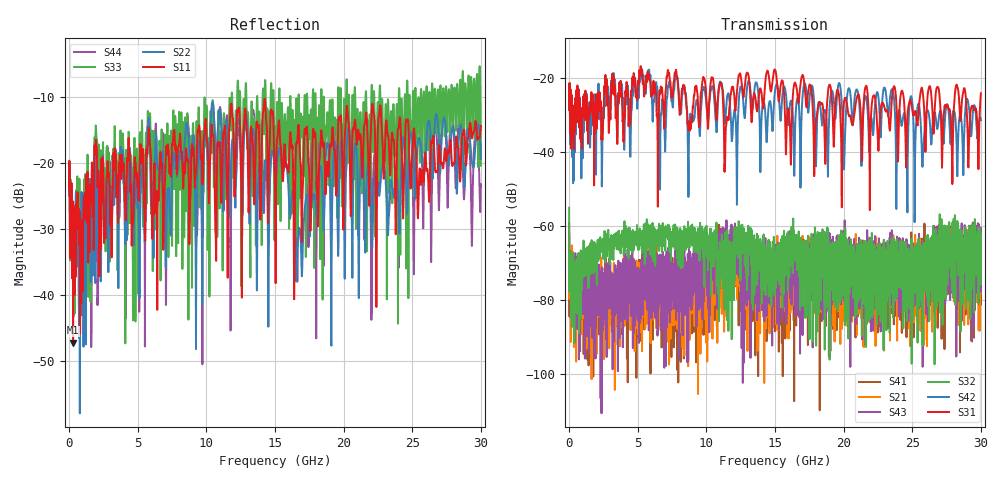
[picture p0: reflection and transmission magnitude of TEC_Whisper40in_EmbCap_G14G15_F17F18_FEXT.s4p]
! Tyco Electronics
! F17F18-G14G15_FEXT
!! PART DESCRIPTION: Whisper 40in Megtron 6 VLP-HVLP-VLP Channel, Embedded Capactior Connecter at one end, bulkhead 2.4mm test pts
!! MODEL DESCRIPTION: System 4-port S-parameter
!! MODEL STATUS: Measured
!! MODEL GEOMETRY: Channel Model
!! MODEL FREQUENCY RANGE: DC to 30.000 GHz in 10.000 MHz frequency steps
!! MODEL EDGE RATE LIMITATION: 12.500 ps (Using conservative 0.5/Fmax rule of thumb)
!! TIME-DOMAIN TRANSFORM CAUTIONS:
!! 1.) Do not simulate transient edge rates faster than the number listed above.  Edge rates faster than this number
!!  contain significant spectral content at frequencies above the model's highest frequency.
!! 2.) Even when simulating edge rates that are slower than the number listed above, be aware that the best time
!!  resolution possible with a direct iFFT is (1 / 2Fmax).  As a result, time resolution is typically not adequate
!!  for most time-domain simulations unless tricks such as windowing are used to minimize leakage and aliasing.
!! 3.) Because the model has a uniform frequency step, a direct iFFT will result in an impulse that that has a time
!!  length given by either (1 / Fstep) or (1 / 2Fstep), depending on the transform being used.  Care has been taken
!!  in selecting the frequency step to ensure a settled impulse response for the model.  Therefore, convolution with
!!  the model's impulse response should present no issues.  However, if directly concatenating s-parameter models
!!  in the frequency domain a user must either interpolate necessary interim frequencies or complete impulse response
!!  zero-padding.  Impulse response zero-padding is more difficult, but more accurate.
!! PORT DEFINITIONS:
!! Port  1  ----->  Side A  F17  G14  Side B  <-----  Port  2
!! Port  3  ----->  Side A  F18  G15  Side B  <-----  Port  4
! Point-to-Point link (differential)  !
! Connectors:  !
!  1: STRADA Whisper  !
! Materials:  !
!  Backplane: Megtron-6 HVLP  !
!  Daughtercard: Megtron-6 VLP  !
! Stack-up:  !
!  Backplane: 20 layers, 200mil thick  !
!  Daughtercard: 14 layers, 110mil thick  !
! Trace Length:  !
!  Backplane: 30in  !
!  Daightercards: 5in  !
! Trace Width:  !
!  Backplane: 7-9-7 mils  !
!  Daughtercards: 6-9-6 mils  !
! Geometry:  !
!  Backplane: Stripline  !
!  Daughtercards: Stripline  !
! Freq. Range: 0 GHz - 30 GHz  !
! Note1: non-mixed-mode s-parameters  !
! Note2: channel includes 2.4mm test points  !
! Touchstone data
! Created: 02-Jul-2013 by IdEM R2011 (7.0.3)
# Hz S MA R 50
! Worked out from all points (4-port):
!   3000 points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, 10 MHz to 30 GHz, reference 50 ohm
!   strongest paths, dB at 10 MHz, 7.51 GHz, 15.01 GHz, 22.51 GHz, 30 GHz:
!     S31: -28.3, -24.8, -17.7, -37.9, -24.0
!     S42: -28.6, -26.2, -23.2, -24.3, -31.3
!     S32: -55.0, -63.8, -70.3, -69.5, -75.7
!     S43: -59.4, -74.1, -69.9, -70.3, -66.4
!     S21: -59.1, -77.9, -76.1, -72.3, -69.5
!     S41: -62.0, -71.7, -76.3, -72.5, -68.9
!   lowest |S11| = -47.2 dB at 300 MHz (marker M1), VSWR 1.01, Z = 49.7 + j0.267 ohm
!   |S11| at or under -10 dB: start of sweep to end of sweep
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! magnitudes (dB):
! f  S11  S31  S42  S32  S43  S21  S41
! 10 MHz  -23.9  -28.3  -28.6  -55.0  -59.4  -59.1  -62.0
! 300 MHz  -47.2  -36.5  -48.4  -84.5  -73.7  -77.7  -72.9
! 10.46 GHz  -15.7  -19.8  -22.2  -63.8  -68.0  -73.8  -67.8
! 11.42 GHz  -16.6  -33.5  -29.6  -65.4  -63.0  -69.9  -66.0
! 12.42 GHz  -12.5  -18.8  -23.8  -61.8  -72.4  -67.7  -77.3
! 16.62 GHz  -17.0  -23.7  -25.4  -66.5  -75.1  -67.0  -67.0
! 30 GHz  -14.4  -24.0  -31.3  -75.7  -66.4  -69.5  -68.9
